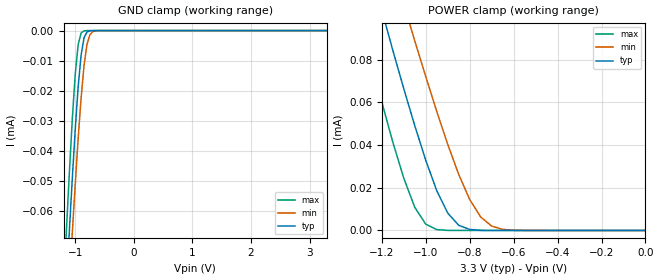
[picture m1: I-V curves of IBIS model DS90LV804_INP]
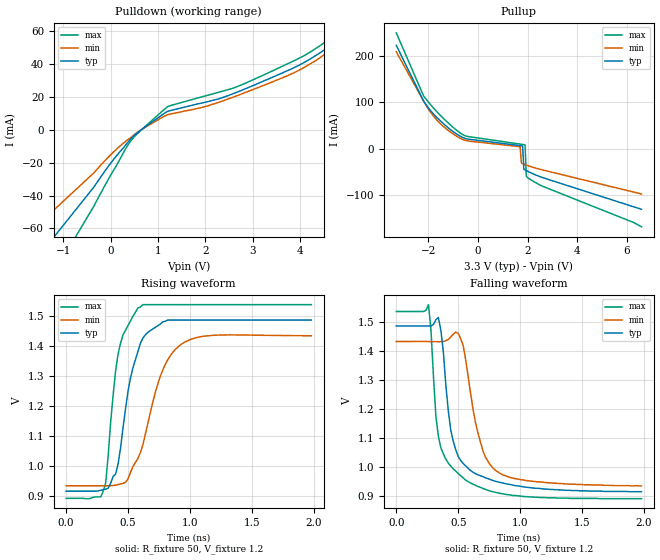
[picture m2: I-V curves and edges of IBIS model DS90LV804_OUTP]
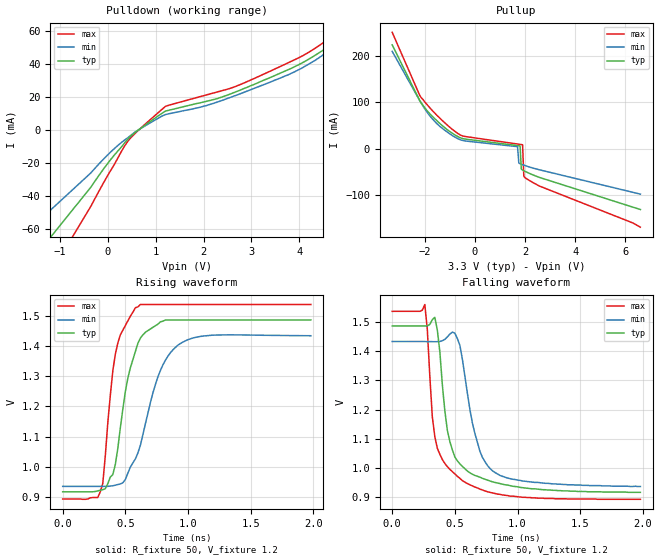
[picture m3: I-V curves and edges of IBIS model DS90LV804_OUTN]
|   National Semiconductor Corporation
|   IBIS Model
|   of
|   DS90LV804TSQ
| 1.5 Gbps 4 Channel LVDS Buffer Repeater
|   with Pre-emphasis
|   32 pin LLP package
[IBIS Ver]   3.2
[Comment Char]   |_char
[File name]   ds90lv804tsq.ibs
[File Rev]   1.2
[Date]   06/14/06
[Source]
|SpectreS simulation
[Notes]
|Created by dglisic
|Rev 1.0   New model;
[Disclaimer]
(C) Copyright National Semiconductor Corporation 2005
   All rights reserved
   National Semiconductor Corporation hereby grants
the user of this IBIS model a non-exclusive, nontransferable
license to use this IBIS model under the following terms.
Before using this IBIS model, the user should read this
license.  If the user does not accept these terms,  the
IBIS model should be returned to National within 30 days.
   The user is granted this license only to use the
IBIS model and is not granted rights to sell, load, rent,
lease or license the IBIS model in whole or in part, or in
modified form to anyone other than user. User may modify
the IBIS model to suit its specific applications but rights
to derivative works and such modifications shall belong to
National.
   This IBIS model is provided on an "AS IS" basis and
National makes absolutely no warranty with respect to the
information contained herein.NATIONAL DISCLAIMS AND CUSTOMER
WAIVES ALL WARRANTIES, EXPRESS OR IMPLIED, INCLUDING
WARRANTIES OF MERCHANTABILITY OR FITNESS FOR A PARTICULAR
PURPOSE. The entire risk as to quality and performance is
with the Customer. ACCORDINGLY, IN NO EVENT SHALL THE
COMPANY BE LIABLE FOR ANY DAMAGES, WHETHER IN CONTRACT OR
TORT,INCLUDING ANY LOST PROFITS OR OTHER INCIDENTAL,
CONSEQUENTIAL, EXEMPLARY, OR PUNITIVE DAMAGES ARISING OUT
OF THE USE OR APPLICATION OF THE IBIS model provided in
this package.Further, National reserves the right to make
changes without notice to any product herein to improve
reliability, function, or design. National does not convey
any license under patent rights or any other intellectual
property rights, including those of third parties.
   National is not obligated to provide maintenance or support
for the licensed IBIS model.
Contact National at ATTN:ENHANCED SOLUTIONS/IBIS MODELS.
5 Foden Road, M/S 01-50, South Porltand, ME 04106
(207) 541-8467
[Copyright]
(c) Copyright 2005 National Semiconductor Corp.
[Component]   DS90LV804
Si_location Pin
Timing_location Pin
[Manufacturer]   National Semiconductor Corp.
[Package]
|   TYP   MIN   MAX
R_pkg   228m   198m   267m
L_pkg   1.39n   1.22n   1.62n
C_pkg   0.0434p   0.0382p   0.0533p
[Pin]   signal_name   model_name   R_pin   L_pin   C_pin
1   GND   GND   243m   1.4908n .0533p
2   GND   GND   229m   1.4025n .0424p
3   VDD   POWER   224m   1.3528n .0390p
4   VDD   POWER   215m   1.3173n .0409p
5   GND   GND   218m   1.3364n .0398p
6   VDD   POWER   232m   1.4032n .0393p
7   VDD   POWER   245m   1.4837n .0406p
8   EN   DS90LV804_CMOSIN   267m   1.6205n .0523p
9   IN0+   DS90LV804_INP   256m   1.5582n .0527p
10   IN0-   DS90LV804_INN   236m   1.4593n .0415p
11   IN1+   DS90LV804_INP   231m   1.3840n .0408p
12   IN1-   DS90LV804_INN   222m   1.3430n .0396p
13   IN2+   DS90LV804_INP   212m   1.3258n .0408p
14   IN2-   DS90LV804_INN   224m   1.2738n .0408p
15   IN3+   DS90LV804_INP   234m   1.4368n .0410p
16   IN3-   DS90LV804_INN   249m   1.5445n .0521p
17   GND   GND   256m   1.5295n .0520p
18   GND   GND   229m   1.3871n .0418p
19   VDD   POWER   220m   1.3194n .0404p
20   VDD   POWER   215m   1.2531n .0395p
21   VDD   POWER   198m   1.2179n .0382p
22   VDD   POWER   206m   1.2347n .0409p
23   NC   NC   219m   1.3000n .0413p
24   NC   NC   227m   1.3843n .0519p
25   OUT3-   DS90LV804_OUTN   256m   1.5372n .0525p
26   OUT3+   DS90LV804_OUTP   232m   1.4194n .0403p
27   OUT2-   DS90LV804_OUTN   215m   1.3437n .0390p
28   OUT2+   DS90LV804_OUTP   204m   1.2922n .0407p
29   OUT1-   DS90LV804_OUTN   213m   1.3089n .0395p
30   OUT1+   DS90LV804_OUTP   218m   1.3511n .0397p
31   OUT0-   DS90LV804_OUTN   215m   1.3974n .0414p
32   OUT0+   DS90LV804_OUTP   239m   1.5121n .0531p
[Series Pin Mapping]   pin_2   model_name
9   10   term_resistor
11   12   term_resistor
13   14   term_resistor
15   16   term_resistor
[Diff Pin] inv_pin   vdiff   tdelay_typ   tdelay_min   tdelay_max
| The '+' pin is Diff_pin and the '-' pin is the inv_pin
| Receiver Vth = +/-100mV
9   10   0.1   0   0   0
11   12   0.1   0   0   0
13   14   0.1   0   0   0
15   16   0.1   0   0   0
26   25   NA   0   0   0
28   27   NA   0   0   0
30   29   NA   0   0   0
32   31   NA   0   0   0
|   Model resistor
[Model]   term_resistor
Model_type   Series
Polarity   Non-Inverting
C_comp   0.0pF   0.0pF   0.0pF
[Temperature Range] 25   85   -40
[Voltage Range]   3.300   3.0   3.6
| Resistance   ohm(typ)   ohm(min)   ohm(max)
[R Series]   100   85   115
| Models and submodels in the file (6): DS90LV804_INP (Input), DS90LV804_INN (Input), DS90LV804_OUTP (Output), DS90LV804_OUTN (Output), DS90LV804_CMOSIN (Input), term_resistor (Series)
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[Model]   DS90LV804_INP
Model_type Input
Vinh=0.05
Vinl=-0.05
C_comp   5pF   5pF   5pF
[Model Spec]
S_overshoot_high   3.3   3.0   3.6
S_overshoot_low   0.0   0.0   0.0
[Temperature Range]   25   85   -40
[Voltage Range]   3.3   3.0   3.6
[GND Clamp]
|V(groundclamp)   I(typ)   I(min)   I(max)
-3.3V     -945.7uA   -911.3uA   -990.7uA
-1.15V    -84.3uA    -101uA     -66uA
-1.1V     -66.3uA    -83.7uA    -47uA
-1.05V    -49uA      -67uA      -29.3uA
-1V       -32.8uA    -51uA      -14.4uA
-950mV    -18.6uA    -35.7uA    -4.63uA
-900mV    -8.13uA    -22.4uA    -803nA
-850mV    -2.42uA    -11.6uA    -85nA
-800mV    -493nA     -4.63uA    -7.57nA
-750mV    -80.3nA    -1.39uA    -657pA
-650mV    -1.78nA    -72.3nA    -4.9pA
3.3V      2.2fA      16fA       2.09fA
[POWER Clamp]
|Vtable   I(typ)   I(min)   I(max)
-3.3V     945.7uA    936uA      962.1uA
-1.3V     141uA      178uA      99.7uA
-1.2V     103uA      141uA      60uA
-1.15V    84.3uA     124uA      41.3uA
-1.1V     66.3uA     106uA      24.4uA
-1.05V    49uA       88.7uA     10.8uA
-1V       32.8uA     72uA       2.92uA
-900mV    8.13uA     40.3uA     40.3nA
-800mV    493nA      14.5uA     307pA
-750mV    80.3nA     6.3uA      26.5pA
-650mV    1.78nA     527nA      201fA
0V        2.2fA      2.73fA     2.22fA
[Model]   DS90LV804_OUTP
Model_type Output
Polarity Non-Inverting
Vref=1.2
Vmeas=1.2
Rref=50   | 100 Ohms Across Outputs OUTP and OUTM
Cref=2p
C_comp   8pF   8pF   8pF
[Temperature Range] 25   85   -40
[Voltage Range]   3.3   3.15   3.45
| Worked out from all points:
|   slope of the pulldown table from 0 to 0.495 V, typ, clamps not added: 29.3 ohm
|   slope of the pullup table from 0 to 0.495 V, typ, clamps not added: 151 ohm
|   falling waveform, R_fixture 50, V_fixture 1.2: 20-80 % time 126ps typ, 147ps min, 123ps max; typ from 1.49 V to 0.916 V
|   rising waveform, R_fixture 50, V_fixture 1.2: 20-80 % time 144ps typ, 207ps min, 102ps max; typ from 0.917 V to 1.49 V
[Pullup]
|Vtable   I(typ)   I(min)   I(max)
-3.3V     223mA      209mA      250mA
-2.2V     103mA      103mA      114mA
-1.6V     64.1mA     58.2mA     76.1mA
-900mV    32.8mA     28mA       41.2mA
1.7V      6.41mA     4.1mA      9.71mA
1.75V     6.07mA     -31mA      9.32mA
1.8V      5.74mA     -32.6mA    8.93mA
1.85V     -44.3mA    -33.6mA    8.54mA
1.9V      -46.2mA    -34.6mA    8.15mA
1.95V     -47.6mA    -35.6mA    -59.6mA
2V        -48.9mA    -36.6mA    -62.7mA
6.6V      -131mA     -98mA      -169mA
[Pulldown]
|V(pulldown)   I(typ)   I(min)   I(max)
-3.3V     -141mA     -105mA     -188.8mA
-358mV    -35mA      -26.3mA    -46.65mA
423mV     -5.55mA    -4.77mA    -6.829mA
1.204V    11.3mA     9.21mA     14.14mA
2.056V    17.2mA     14.6mA     21.07mA
2.624V    22.4mA     20.3mA     25.75mA
3.902V    38.2mA     35.1mA     42.43mA
4.541V    49.1mA     46.5mA     53.61mA
4.683V    52.1mA     51.3mA     56.65mA
4.896V    57.4mA     63.7mA     61.48mA
5.038V    62.9mA     74.8mA     65.14mA
6.6V      227mA      228mA      232.6mA
[Falling Waveform]
R_fixture=50
V_fixture=1.2
V_fixture_min=1.2
V_fixture_max=1.2
0s        1.487V     1.434V     1.537V
260ps     1.487V     1.434V     1.561V
320ps     1.509V     1.433V     1.175V
340ps     1.517V     1.433V     1.107V
440ps     1.129V     1.45V      1.004V
500ps     1.037V     1.462V     979mV
560ps     1.005V     1.372V     956mV
660ps     974mV      1.118V     934mV
800ps     952mV      990mV      914mV
1.98ns    916mV      936mV      892mV
[Rising Waveform]
R_fixture=50
V_fixture=1.2
V_fixture_min=1.2
V_fixture_max=1.2
0s        917mV      935mV      893mV
300ps     922mV      935mV      917mV
320ps     924mV      935mV      945mV
380ps     966mV      936mV      1.237V
420ps     1.008V     939mV      1.374V
500ps     1.25V      958mV      1.468V
580ps     1.382V     1.026V     1.527V
760ps     1.473V     1.299V     1.538V
920ps     1.487V     1.403V     1.538V
1.98ns    1.487V     1.435V     1.538V
[Ramp]
|   typ   min   max
dV/dt_r   320mV/.213ns   310mV/.222ns   330mV/.150ns
dV/dt_f   320mv/.192ns   310mv/.241ns   330mv/.156ns
R_load=50
|[End   DS90LV804_OUTP
[Model]   DS90LV804_OUTN
Model_type Output
Polarity Inverting
Vref=1.2
Vmeas=1.2
Rref=50   | 100 Ohms Across Outputs OUTP and OUTM
Cref=2p
C_comp   8pF   8pF   8pF
[Temperature Range] 25   85   -40
[Voltage Range]   3.3   3.15   3.45
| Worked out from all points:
|   slope of the pulldown table from 0 to 0.495 V, typ, clamps not added: 29.3 ohm
|   slope of the pullup table from 0 to 0.495 V, typ, clamps not added: 151 ohm
|   falling waveform, R_fixture 50, V_fixture 1.2: 20-80 % time 126ps typ, 147ps min, 123ps max; typ from 1.49 V to 0.916 V
|   rising waveform, R_fixture 50, V_fixture 1.2: 20-80 % time 144ps typ, 207ps min, 102ps max; typ from 0.917 V to 1.49 V
[Pullup]
|Vtable   I(typ)   I(min)   I(max)
-3.3V     223mA      209mA      250mA
-2.2V     103mA      103mA      114mA
-1.6V     64.1mA     58.2mA     76.1mA
-900mV    32.8mA     28mA       41.2mA
1.7V      6.41mA     4.1mA      9.71mA
1.75V     6.07mA     -31mA      9.32mA
1.8V      5.74mA     -32.6mA    8.93mA
1.85V     -44.3mA    -33.6mA    8.54mA
1.9V      -46.2mA    -34.6mA    8.15mA
1.95V     -47.6mA    -35.6mA    -59.6mA
2V        -48.9mA    -36.6mA    -62.7mA
6.6V      -131mA     -98mA      -169mA
[Pulldown]
|V(pulldown)   I(typ)   I(min)   I(max)
-3.3V     -141mA     -105mA     -188.8mA
-358mV    -35mA      -26.3mA    -46.65mA
423mV     -5.55mA    -4.77mA    -6.829mA
1.204V    11.3mA     9.21mA     14.14mA
2.056V    17.2mA     14.6mA     21.07mA
2.624V    22.4mA     20.3mA     25.75mA
3.902V    38.2mA     35.1mA     42.43mA
4.541V    49.1mA     46.5mA     53.61mA
4.683V    52.1mA     51.3mA     56.65mA
4.896V    57.4mA     63.7mA     61.48mA
5.038V    62.9mA     74.8mA     65.14mA
6.6V      227mA      228mA      232.6mA
[Falling Waveform]
R_fixture=50
V_fixture=1.2
V_fixture_min=1.2
V_fixture_max=1.2
0s        1.487V     1.434V     1.537V
260ps     1.487V     1.434V     1.561V
320ps     1.509V     1.433V     1.175V
340ps     1.517V     1.433V     1.107V
440ps     1.129V     1.45V      1.004V
500ps     1.037V     1.462V     979mV
560ps     1.005V     1.372V     956mV
660ps     974mV      1.118V     934mV
800ps     952mV      990mV      914mV
1.98ns    916mV      936mV      892mV
[Rising Waveform]
R_fixture=50
V_fixture=1.2
V_fixture_min=1.2
V_fixture_max=1.2
0s        917mV      935mV      893mV
300ps     922mV      935mV      917mV
320ps     924mV      935mV      945mV
380ps     966mV      936mV      1.237V
420ps     1.008V     939mV      1.374V
500ps     1.25V      958mV      1.468V
580ps     1.382V     1.026V     1.527V
760ps     1.473V     1.299V     1.538V
920ps     1.487V     1.403V     1.538V
1.98ns    1.487V     1.435V     1.538V
[Ramp]
|   typ   min   max
dV/dt_r   320mV/.213ns   310mV/.222ns   330mV/.150ns
dV/dt_f   320mv/.192ns   310mv/.241ns   330mv/.156ns
R_load=50
|[End   DS90LV804_OUTN
